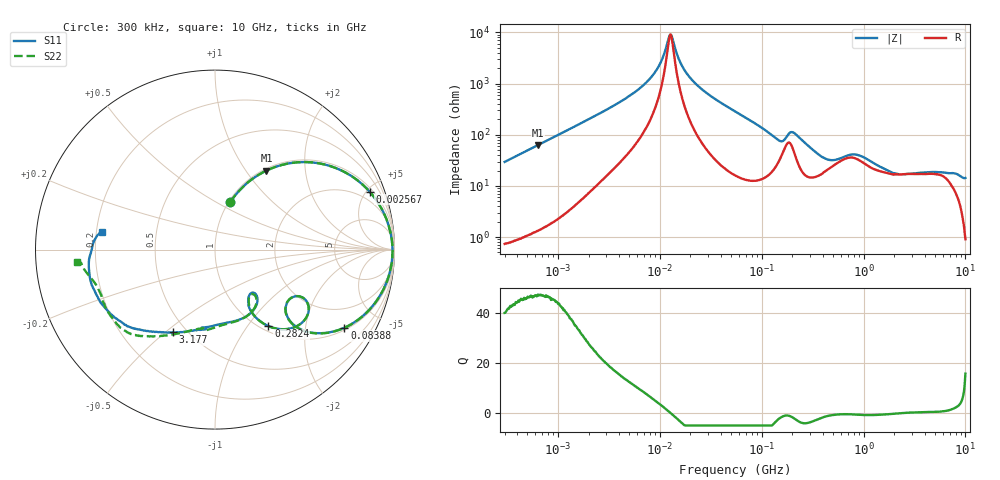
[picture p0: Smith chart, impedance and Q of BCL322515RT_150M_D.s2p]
! S-Parameter Data Generated by TDK Corporation
! Copyright(C) 2024 TDK Corporation.
! All Rights Reserved.
! TDK P/N: BCL322515RT-150M-D (SMD / SMT Inductor (Coil))
! Property: L=15uH at 1MHz
! Size(LxWxT): 3.2x2.5x1.5mm
! Model Type: s2p (Touchstone File Format Version 1.0)
! Frequency: DC=Yes Start=0.3MHz Stop=10000MHz 802points Log-sweep
! Model Generated on May 28, 2024
! Terms and conditions regarding TDK Simulation Models:
! 1)This simulation model is being provided solely for informational
!  purposes. Please refer to the specifications of the products in
!  terms of detailed characteristics of such products.
! 2)In no event shall TDK Corporation of any of its subsidiaries be
!  liable for any loss or damage arising, directly or indirectly,
!  from any information contained in this simulation model, including,
!  but not limited to loss or damages arising from any inaccuracies,
!  omissions or errors in connection with such information.
! 3)Any and all copyrights on this simulation model are owned by
!  TDK Corporation.  Duplication or redistribution of this simulation
!  model without prior written permission from TDK Corporation
!  is prohibited.
! 4)This simulation model is subject to any modification or change
!  without any prior notice.
! 5)Neither TDK Corporation nor any of its subsidiaries shall make any
!  warranty, express or implied, including but not limited to the
!  correctness, implied warranties of merchantability and fitness for
!  a particular purpose with respect to this simulation models.
! 6)The use of this simulation model shall be deemed to have consented
!  to the terms and conditions hereof.
! Port Assignments:
!  1 ---@@@--- 2
! Applicable Conditions:
!  Temperature = 25 degC
!  DC Bias Current = 0 A
!  Small Signal Operation
# Hz S MA R 50
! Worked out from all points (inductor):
!   801 points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, 300 kHz to 10 GHz, reference 50 ohm
!   read as one part in series: L = 15.6 uH near 318.3 kHz
!   highest Q = 47.1 at 636.7 kHz (marker M1), where L = 15.7 uH
!   self-resonance near 12.73 MHz
!   S11 on the Smith chart (normalised r, x): 300 kHz: 1.02, +0.59; 2.567 MHz: 1.24, +5.22; 83.88 MHz: 1.09, -3.25; 282.4 MHz: 1.08, -1.26; 3.177 GHz: 0.42, -0.53; 10 GHz: 0.22, +0.07
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300000  0.2787 72.1  0.9532 -16.5  0.9531 -16.4  0.2789 72.1
636701  0.5253 56.9  0.8397 -31.8  0.8398 -31.8  0.5252 57.0
1713600  0.8507 29.8  0.4988 -58.3  0.499 -58.3  0.8508 29.8
2566584  0.9197 20.6  0.3535 -66.9  0.3536 -66.8  0.9198 20.6
6041662  0.9784 7.3  0.1316 -77.0  0.1317 -77.0  0.9784 7.3
9671944  0.9874 2.3  0.04695 -73.6  0.04697 -73.6  0.9877 2.3
1.289893e7  0.989 -0.5  0.01101 9.7  0.01101 9.7  0.9893 -0.5
1.603896e7  0.9885 -2.6  0.03951 71.7  0.03953 71.7  0.9887 -2.7
2.036513e7  0.9859 -5.2  0.08053 77.1  0.08055 77.1  0.9861 -5.2
5.477226e7  0.9286 -20.3  0.3226 66.4  0.3227 66.4  0.9288 -20.4
8.38787e7  0.8418 -31.1  0.4825 54.7  0.4827 54.7  0.8418 -31.2
1.437797e8  0.5575 -43.1  0.667 27.6  0.6672 27.6  0.5568 -43.3
1.743231e8  0.5246 -29.6  0.5673 17.6  0.5675 17.6  0.5234 -29.7
2.039737e8  0.6311 -35.1  0.5448 28.6  0.5451 28.6  0.6308 -35.1
2.824321e8  0.5199 -55.0  0.7475 22.4  0.7478 22.4  0.5213 -55.0
3.126428e8  0.4672 -58.0  0.7766 18.0  0.777 18.0  0.4694 -57.9
5.745924e8  0.321 -48.3  0.7465 -2.6  0.7467 -2.6  0.325 -49.8
1.767019e9  0.4284 -93.1  0.7509 -23.0  0.7511 -23.0  0.438 -91.6
3.177248e9  0.5177 -117.0  0.6768 -46.9  0.677 -46.9  0.5266 -116.2
6.41458e9  0.6761 -146.1  0.5013 -78.5  0.5015 -78.7  0.6874 -146.0
8.211115e9  0.713 -168.6  0.4404 -99.0  0.441 -99.1  0.7001 -165.6
1e10  0.6398 171.1  0.3457 -111.6  0.3454 -111.7  0.771 -174.8
